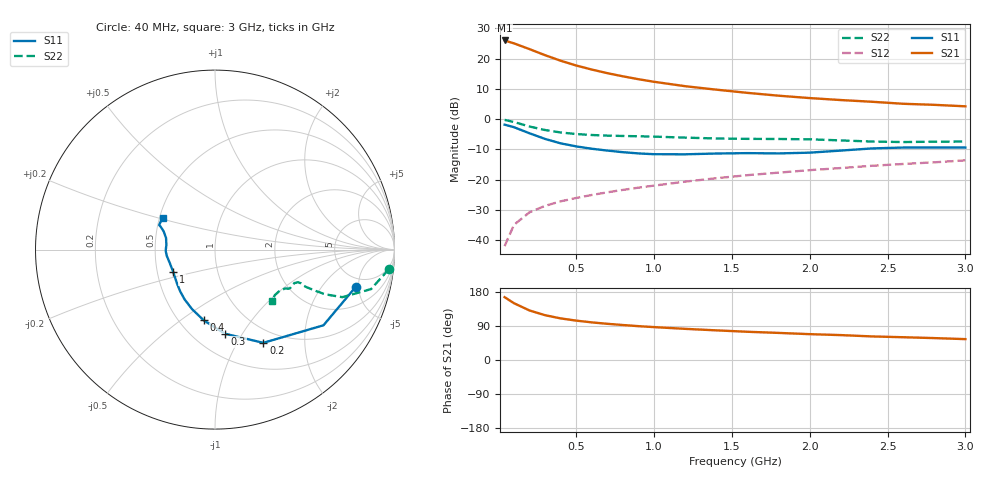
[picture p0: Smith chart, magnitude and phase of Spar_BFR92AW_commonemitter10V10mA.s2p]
! Filename:  BFR92AWH.S2P  Version:  4.0
! NXP part #: BFR92AW  Date: Jun 1994
! Bias condition: Vce=10V, Ic=10mA
#  MHz  S  MA  R  50
! Freq  S11  S21  S12  S22  !GUM [dB]
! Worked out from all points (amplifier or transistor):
!   21 points, 40 MHz to 3 GHz, reference 50 ohm
!   highest |S21| = 26.0 dB at 40 MHz (marker M1)
!   |S21| within 3 dB of that: start of sweep to 206.9 MHz
!   unconditionally stable (mu >= 1): 759.1 MHz to end of sweep
!   at 300 MHz: K = 0.65, MSG = 24.9 dB, |S12| = -28.6 dB
!   at 1 GHz: K = 1.08, MAG = 15.4 dB, |S12| = -21.9 dB
!   at 3 GHz: K = 1.10, MAG = 7.0 dB, |S12| = -13.6 dB
!   lowest NFmin = 2.00 dB at 500 MHz
!   S11 on the Smith chart (normalised r, x): 40 MHz: 3.85, -4.66; 200 MHz: 0.82, -1.29; 300 MHz: 0.70, -0.84; 400 MHz: 0.65, -0.61; 1 GHz: 0.61, -0.16; 3 GHz: 0.52, +0.21
40  0.812 -14.7  19.94 165.8  0.008 82.0  0.974 -6.5
100  0.737 -34.9  17.86 149.9  0.018 71.8  0.897 -14.2
200  0.585 -62.6  14.35 130.7  0.029 63.5  0.757 -20.5
300  0.472 -83.2  11.39 118.2  0.037 60.4  0.662 -22.1
400  0.399 -99.1  9.23 109.8  0.044 60.7  0.603 -22.3
500  0.355 -111.2  7.695 103.9  0.05 62.0  0.568 -22.3
600  0.325 -121.4  6.595 99.3  0.056 64.1  0.548 -22.3
700  0.303 -129.8  5.752 95.5  0.062 65.4  0.535 -22.1
800  0.285 -137.6  5.099 92.3  0.068 66.7  0.528 -21.9
900  0.272 -144.8  4.568 89.3  0.074 67.7  0.522 -21.6
1000  0.264 -151.7  4.144 86.8  0.08 68.8  0.515 -21.4
1200  0.263 -164.0  3.504 82.2  0.093 70.2  0.496 -21.5
1400  0.271 -172.6  3.072 78.2  0.106 71.5  0.48 -22.9
1600  0.275 -178.8  2.719 74.5  0.119 72.0  0.473 -25.5
1800  0.272 174.8  2.442 71.5  0.131 73.1  0.471 -27.0
2000  0.28 166.8  2.23 68.2  0.144 73.6  0.465 -27.9
2200  0.303 160.5  2.069 65.7  0.156 74.1  0.446 -29.1
2400  0.329 157.1  1.939 62.2  0.17 74.3  0.427 -32.5
2600  0.34 156.3  1.796 60.1  0.182 74.3  0.419 -37.2
2800  0.34 153.9  1.725 57.8  0.194 75.1  0.425 -40.6
3000  0.34 149.1  1.63 55.1  0.209 75.2  0.427 -42.5
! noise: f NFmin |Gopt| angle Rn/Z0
500  2  0.385  17.8  0.42
1000  2.5  0.271  47.4  0.45
2000  3.4  0.165  167.6  0.3
